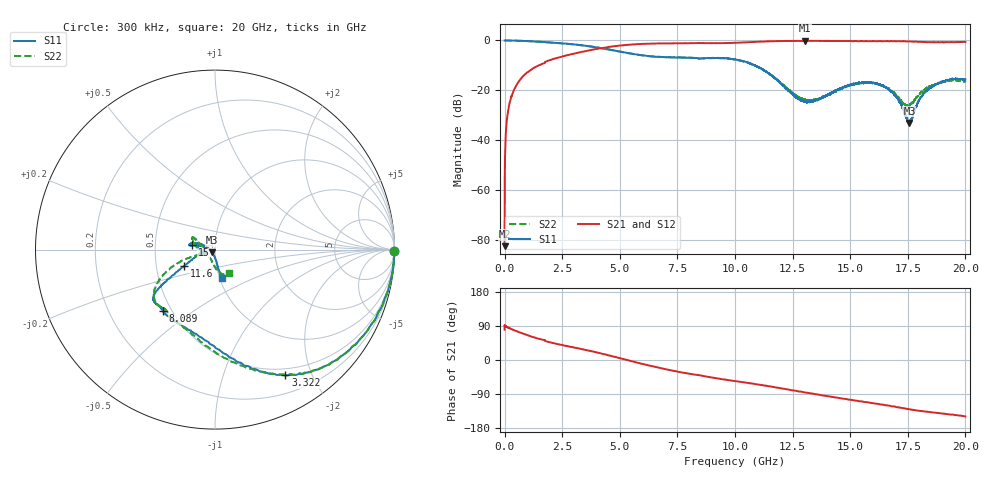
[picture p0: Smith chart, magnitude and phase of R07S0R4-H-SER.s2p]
!{R07S0R4}
!Johanson Technology Inc.
!www.johansontechnology.com
!Test Board Conditions:
!Substrate Type  RO4350B
!Substrate Thickness  10 mil
!Substrate Dk  3.66
!TL Type: GCPW
!TL Trace Width  21 mil
!TL Gap  20 mil
!Electrode orientation  Horizontal
!DUT TOPOLOGY	SERIES
!Mounting Pad LxW  16x21 mil
! Created Fri Feb  5 23:02:21 2021
# hz S ma R 50
! 2 Port Network Data from SP1.SP block
! freq  magS11  angS11  magS21  angS21  magS12  angS12  magS22  angS22
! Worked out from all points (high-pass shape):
!   20001 points, 300 kHz to 20 GHz, reference 50 ohm
!   highest |S21| = -0.13 dB at 13.03 GHz (marker M1); lowest = -82.5 dB at 300 kHz (marker M2)
!   |S21| within 3 dB of the highest: 4.173376 GHz to 4.175283 GHz (1.907 MHz wide, 0.0457 % of centre); 4.177 GHz to end of sweep
!   lowest |S11| = -33.1 dB at 17.57 GHz (marker M3), VSWR 1.05, Z = 48.4 - j1.42 ohm
!   |S11| at or under -10 dB: 10.85688 GHz to 10.85756 GHz (677.7 kHz wide, 0.00624 % of centre); 10.85923 GHz to 10.86076 GHz (1.53 MHz wide, 0.0141 % of centre); 10.87 GHz to end of sweep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
!   |S22| runs from -26.5 to 0.0 dB; largest |S21 - S12| = 0.011
!   S11 on the Smith chart (normalised r, x): 300 kHz: open; 3.322 GHz: 0.41, -1.63; 8.089 GHz: 0.45, -0.39; 11.6 GHz: 0.70, -0.13; 15 GHz: 0.77, +0.04; 20 GHz: 1.02, -0.34
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300000  1 -0.6  7.494e-05 80.0  0.0001402 80.0  0.9991 -0.5
1.013e8  0.9974 -2.7  0.02602 87.1  0.02595 87.2  0.998 -2.7
1.343e8  0.999 -3.6  0.03448 86.0  0.03447 86.3  0.9994 -3.6
2.683e8  0.9964 -7.1  0.06846 82.6  0.06848 82.5  0.9968 -7.1
5.003e8  0.9904 -13.0  0.1238 76.6  0.1237 76.5  0.9913 -13.0
1.3643e9  0.9498 -31.7  0.2971 58.0  0.297 58.1  0.9498 -31.5
3.3223e9  0.803 -60.7  0.5882 29.1  0.5867 29.1  0.8055 -60.3
3.3343e9  0.8022 -60.9  0.5898 28.9  0.5882 28.9  0.8041 -60.4
5.1903e9  0.5782 -85.5  0.8052 1.9  0.8063 1.9  0.5763 -89.3
6.6673e9  0.47 -108.7  0.872 -20.1  0.8718 -20.1  0.4709 -110.5
8.0893e9  0.4497 -130.1  0.8818 -36.8  0.8822 -36.8  0.4494 -122.7
1.00003e10  0.4184 -143.7  0.8965 -55.6  0.8988 -55.6  0.4126 -145.6
1.16033e10  0.1954 -152.2  0.9643 -70.5  0.9654 -70.5  0.1984 -161.3
1.30263e10  0.06149 177.8  0.9852 -85.6  0.9841 -85.4  0.06455 -158.5
1.33343e10  0.05859 167.4  0.9809 -88.6  0.9816 -88.6  0.06196 -159.0
1.50003e10  0.1289 169.2  0.978 -104.9  0.9759 -104.8  0.1267 162.6
1.59433e10  0.142 167.0  0.9699 -113.5  0.9692 -113.6  0.1402 151.6
1.66673e10  0.1049 161.2  0.9645 -120.3  0.9679 -120.4  0.1084 154.9
1.75703e10  0.02212 -138.3  0.957 -129.9  0.9582 -129.9  0.04793 -133.9
1.80093e10  0.0655 -83.3  0.9381 -134.0  0.9384 -134.2  0.08291 -94.6
1.84673e10  0.1112 -79.4  0.9227 -137.5  0.9234 -137.5  0.1202 -82.6
2e10  0.164 -76.8  0.9394 -148.8  0.937 -148.7  0.1524 -58.6
